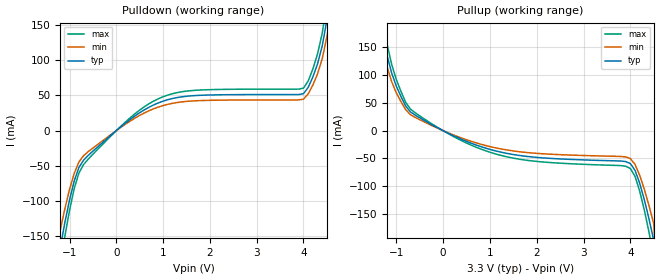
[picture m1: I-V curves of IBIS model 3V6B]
[IBIS Ver]   2.1
[File name]   581-01_3.ibs
[File Rev]   2.0
[Date]   1/20/00
[Source]   ICS MicroClock Applications Engineering 2
[Disclaimer] This information is for modeling purposes only, and is
(C) Copyright Integrated Circuit Systems, Inc. 1997-2001
   All rights reserved
ICS hereby grants the user of this IBIS model a non-exclusive,
nontransferable license to use this IBIS model under the following terms.
Before using this IBIS model, the user should read this license.
If the user does not accept these terms,  the IBIS model should be
returned to ICS within 30 days.
   The user is granted this license only to use the IBIS model and
is not granted rights to sell, load, rent, lease or license the IBIS
model in whole or in part, or in modified form to anyone other than
user. User may modify the IBIS model to suit its specific
applications but rights to derivative works and such modifications
shall belong to ICS.
   This IBIS model is provided on an "AS IS" basis and ICS makes
absolutely no warranty with respect to the information contained
herein. ICS DISCLAIMS AND CUSTOMER WAIVES ALL WARRANTIES, EXPRESS
OR IMPLIED, INCLUDING WARRANTIES OF MERCHANTABILITY OR FITNESS FOR
A PARTICULAR PURPOSE. The entire risk as to quality and performance
is with the Customer. ACCORDINGLY, IN NO EVENT SHALL THE COMPANY BE
LIABLE FOR ANY DAMAGES, WHETHER IN CONTRACT OR TORT,INCLUDING ANY
LOST PROFITS OR OTHER INCIDENTAL, CONSEQUENTIAL, EXEMPLARY, OR
PUNITIVE DAMAGES ARISING OUT OF THE USE OR APPLICATION OF THE IBIS
model provided in this package. Further, ICS reserves the right to
make changes without notice to any product herein to improve
reliability, function, or design. ICS does not convey any license
under patent rights or any other intellectual property rights,
including those of third parties.
   ICS is not obligated to provide maintenance or support
for the licensed IBIS model.
[Component]   ICS581-01
[Manufacturer] Integrated Circuit Systems Inc.
[Package]
|   typ   min   max
R_pkg   40m   35m   45m
L_pkg   1.65nH   1.35nH   1.95nH
C_pkg   0.24pF   0.14pF   0.34pF
[pin]   signal_name   model_name   R_pin   L_pin   C_pin
   14   CLK1   3V6B
   13   CLK2   3V6B
   12   CLK3   3V6B
   11   CLK4   3V6B
| Models and submodels in the file (1): 3V6B (Output)
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|   ICS581-01,-02 3.3V Clock Drive Model
| This model is suitable for all 1X output pins on the
| ICS581 family
[Model]   3V6B
Model_type   Output
Polarity   Non-Inverting
|   typ   min   max
C_comp   5pF   4pF   6pF
|   typ   min   max
[Voltage range]  3.3V   3.15V   3.45V
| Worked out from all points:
|   slope of the pulldown table from 0 to 0.495 V, typ, clamps not added: 19.7 ohm
|   slope of the pullup table from 0 to 0.495 V, typ, clamps not added: 26 ohm
[pulldown]
|Voltage I (typ)   I (min)   I (max)
-3.3V     -3A        -3A        -3A
-1.3V     -199.8mA   -169.9mA   -229.8mA
-1.2V     -166.8mA   -141.8mA   -191.8mA
-1.1V     -130.6mA   -111mA     -150.2mA
-900mV    -71.6mA    -60.86mA   -82.34mA
-700mV    -41.99mA   -35.69mA   -48.29mA
900mV     39.17mA    33.3mA     45.05mA
4V        52.21mA    44.38mA    60.04mA
4.4V      119.6mA    101.7mA    137.6mA
4.5V      156.3mA    132.9mA    179.8mA
4.6V      199.2mA    169.3mA    229.1mA
6.6V      3A         3A         3A
[pullup]
|Voltage I (typ)   I (min)   I (max)
-3.3V     3A         3A         3A
-1.4V     199.6mA    169.7mA    229.6mA
-1.3V     177.1mA    150.6mA    203.7mA
-1V       79.39mA    67.48mA    91.3mA
-800mV    43.9mA     37.32mA    50.49mA
-600mV    27.85mA    23.68mA    32.03mA
1.2V      -38.21mA   -32.47mA   -43.94mA
4V        -59.36mA   -50.46mA   -68.26mA
4.2V      -94.82mA   -80.6mA    -109mA
4.4V      -159.4mA   -135.5mA   -183.3mA
4.5V      -197.4mA   -167.8mA   -227mA
6.6V      -3A        -3A        -3A
[Ramp]
|   typ   min   max
dV/dt_r   1.24/0.57n   1.17/0.63n   1.30/0.52n
dV/dt_f   1.35/0.79n   1.28/0.87n   1.42/0.71n
